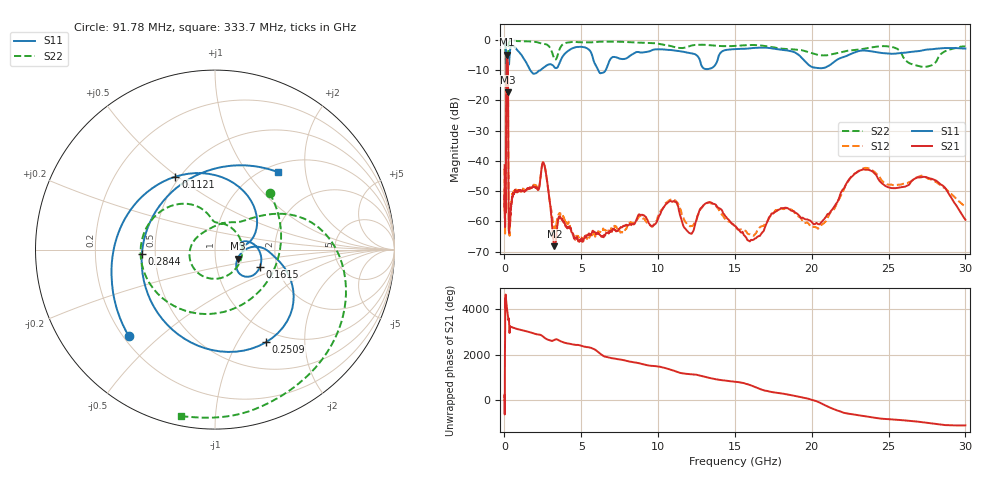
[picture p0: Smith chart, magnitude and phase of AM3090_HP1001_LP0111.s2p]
! Date/Time: Thu, Feb 28, 2019 2:03 PM
! Network Analyzer: Agilent Technologies E8364B Rev: A.07.50.67
! Sweep from 0.010 to 30.000 GHz, 1601 Points, Sweep Type: LOG
! Power Supply: 5.023 V, 0.002 A
# Hz S DB R 50
!freq MagS11 AngS11 MagS21 AngS21 MagS12 AngS12 MagS22 AngS22
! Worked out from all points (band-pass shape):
!   1601 points, 10 MHz to 30 GHz, reference 50 ohm
!   highest |S21| = -4.84 dB at 166.5 MHz (marker M1); lowest = -68.2 dB at 3.253 GHz (marker M2)
!   |S21| within 3 dB of the highest: 124.6 MHz to 219.9 MHz (95.25 MHz wide, 55.3 % of centre)
!   lowest |S11| = -17.3 dB at 199.3 MHz (marker M3), VSWR 1.31, Z = 64 - j6.64 ohm
!   |S11| at or under -10 dB: 120.7 MHz to 222.8 MHz (102.1 MHz wide, 59.5 % of centre); 1.678 GHz to 2.352 GHz (673.8 MHz wide, 33.4 % of centre); 6.099 GHz to 6.59 GHz (491 MHz wide, 7.74 % of centre)
!   |S22| runs from -18.7 to -0.2 dB; largest |S21 - S12| = 0.015
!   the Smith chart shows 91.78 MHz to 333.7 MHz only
!   S11 on the Smith chart (normalised r, x): 91.78 MHz: 0.22, -0.40; 112.1 MHz: 0.48, +0.49; 161.5 MHz: 1.62, -0.34; 250.9 MHz: 0.84, -1.32; 284.4 MHz: 0.42, -0.02; 333.7 MHz: 1.13, +1.41
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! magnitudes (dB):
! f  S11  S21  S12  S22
! 10 MHz  -0.2  -41.4  -43.1  -0.6
! 38.04 MHz  -0.5  -58.7  -60.5  -1.4
! 91.78 MHz  -3.3  -48.5  -47.6  -7.2
! 112.1 MHz  -6.7  -17.9  -17.9  -7.7
! 144.7 MHz  -13.2  -5.2  -5.1  -16.4
! 161.5 MHz  -11.4  -4.9  -4.8  -16.1
! 166.5 MHz  -11.5  -4.8  -4.8  -15.9
! 199.3 MHz  -17.3  -5.5  -5.5  -18.7
! 228.2 MHz  -8.9  -10.5  -10.5  -12.2
! 250.9 MHz  -4.6  -33.5  -33.6  -3.0
! 284.4 MHz  -7.8  -60.7  -63.6  -1.0
! 333.7 MHz  -5.1  -60.7  -64.7  -0.5
! 550.5 MHz  -2.0  -50.7  -51.2  -0.3
! 2.084 GHz  -10.9  -48.9  -48.4  -0.7
! 2.597 GHz  -9.0  -41.3  -41.2  -1.3
! 3.253 GHz  -9.0  -68.2  -62.2  -6.4
! 7.926 GHz  -6.1  -61.1  -62.5  -0.7
! 13.4 GHz  -9.5  -53.7  -54.0  -1.8
! 16.21 GHz  -2.7  -66.1  -64.8  -1.7
! 20.61 GHz  -9.4  -60.4  -61.2  -5.1
! 23.36 GHz  -3.5  -42.8  -42.5  -3.0
! 30 GHz  -2.9  -59.5  -54.9  -2.1
